ORGANIZATION_BLOCK MAIN:OB1
TITLE= Inversione di Marcia di un M.A.T
// Simulatore: 01
// Versione: 1.0
// DATA: 26/02/2002
//
//***DESCRIZIONE***
// Il motore viene inserito tramite il pulsante SB2
// per il funzionamento in "Marcia Avanti", e SB3  per
// la "Marcia Indietro".
// Il Pulsante SB1  viene usato per arrestare la marcia
// del motore in qualsiasi momento.
// Il motore può essere commutato direttamente da uno all'altro
// senso di marcia senza che esso debba essere disinserito
// mediante il pulsante di arresto SB1.
//
// Per motivi di sicurezza un contatto NC del Relè Termico FR
// viene collegato, in hardware, a monte delle bobine dei contattori
// in modo da consentire la sicura diseccitazione dei contattori
// stessi in caso di intervento della protezione.
// Un contatto NC di RT viene però riportato anche su un ingresso
// del PLC per disattivare le uscite del PLC in caso
// di intervento dello stesso e segnalarne lo stato mediante la
// lampada di segnalazione HL4.
//
// Oltre all'interblocco hardware per impedire l'eccitazione
// contemporanea dei due contattori (sempre indispensabile!) il
// programma ne effettua anche uno software  interrogando lo
// stato delle uscite dei contattori KM1 e KM2.
//
// Il programma è stato svolto con il metodo delle memorie
// con SET/RESET.
//
//

BEGIN
NETWORK 1 //Gestione SET Marcia Indietro Motore
//
LD I0.3
S Q0.0 1

NETWORK 2 //Gestione Reset Marcia Indietro
//
LDN I0.1
O I0.2
O Q0.1
ON I0.5
R Q0.0 1

NETWORK 3 //Gestione SET Marcia Avanti Motore
//
LD I0.2
S Q0.1 1

NETWORK 4 //Gestione RESET Marcia Avanti
//
LDN I0.1
O I0.3
ON I0.5
O Q0.0
R Q0.1 1

NETWORK 5 //Segnalazione motore fermo
//
LDN Q0.0
AN Q0.1
= Q0.2

NETWORK 6 //Segnalazione Marcia Avanti
//
LD Q0.1
= Q0.3

NETWORK 7 //Segnalazione Marcia indietro
//
LD Q0.0
= Q0.4

NETWORK 8 //Segalazione Relè Termico scattato
//
LDN I0.5
= Q0.5

END_ORGANIZATION_BLOCK

